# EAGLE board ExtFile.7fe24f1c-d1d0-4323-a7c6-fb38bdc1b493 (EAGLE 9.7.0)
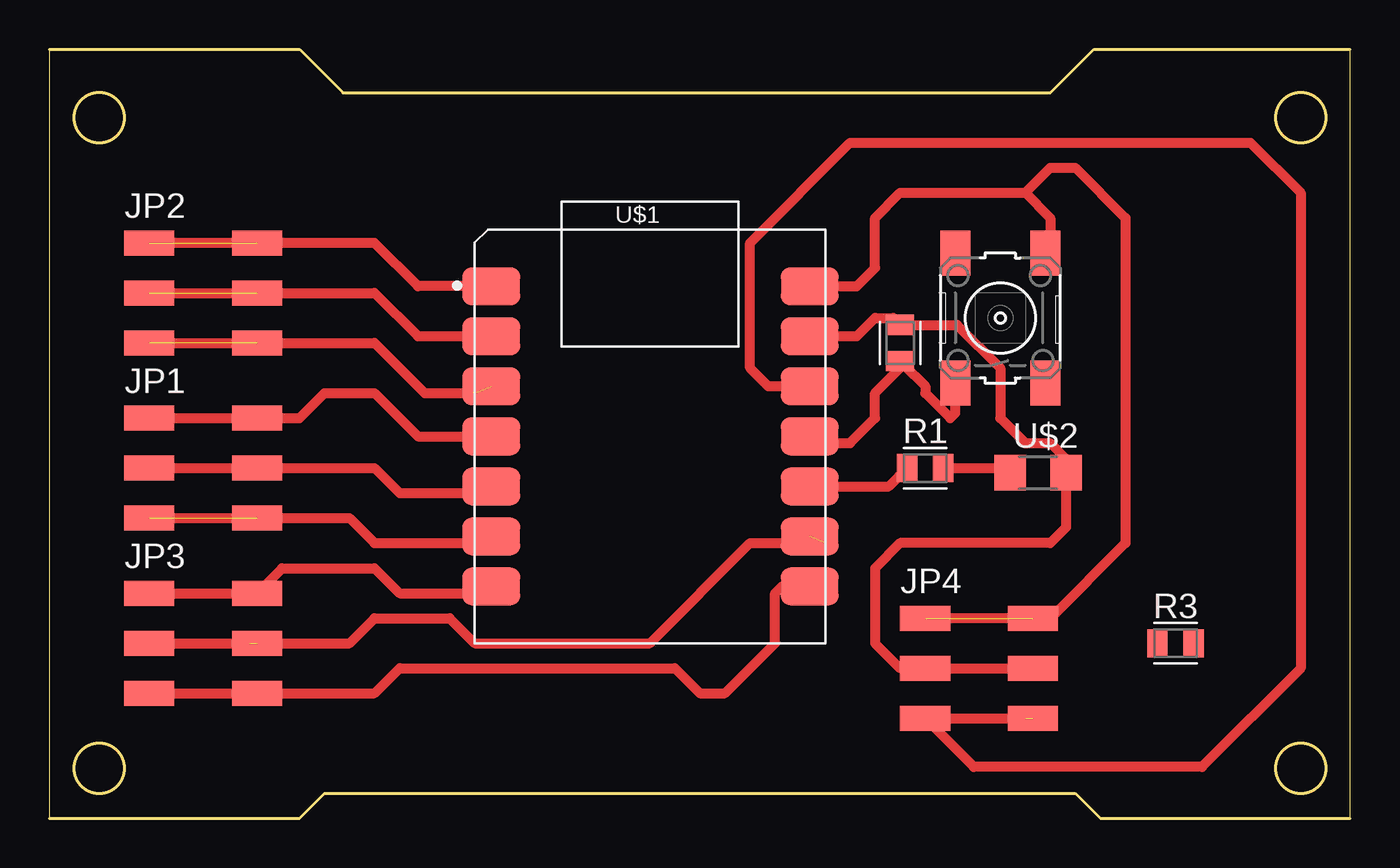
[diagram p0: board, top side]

Size 66.02 x 39.04 mm. Coordinates in mm from the lower left corner, seen from the top.
Outline: 66.02,0 66.02,39.04 53.01,39.04 50.8,36.83 14.91,36.83 12.7,39.04 0,39.04 0,0 12.7,0 13.97,1.27 52.07,1.27 53.34,0 66.02,0
Outline: circle at 2.54,35.56 radius 1.27
Outline: circle at 2.54,2.54 radius 1.27
Outline: circle at 63.5,35.56 radius 1.27
Outline: circle at 63.5,2.54 radius 1.27
Outline: circle at 63.5,35.56 radius 1.27
Outline: circle at 2.54,2.54 radius 1.27
Outline: circle at 63.5,2.54 radius 1.27
Copper layers (1*16): Top / Bottom
Stack-up Default Layer Stack: Top SilkScreen Epoxy Ink / Top SolderMask SR:Green 0.0254mm Dk 4.3 / Top Surface Finish Lead-Free 0.02mm / Top CuFoil:007 0.035mm / Dielectric-1 User Defined 1.5mm / Bottom CuFoil:007 0.035mm / Bottom Surface Finish Lead-Free 0.02mm / Bottom SolderMask SR:Green 0.0254mm Dk 4.3 / Bottom SilkScreen Epoxy Ink
Design rules: minimum drill size 0.35mm, minimum copper width 6mil, keepout clearance 0mil, drill distance 6mil, via restrict clearance 0mil, solder-mask clearance 0mil, dimension clearance 40mil, restrict clearance 0mil, copper clearance wire_polygon to wire_polygon 6mil, copper clearance wire_polygon to pad_smd 6mil, copper clearance wire_polygon to via 6mil, copper clearance pad_smd to pad_smd 6mil, copper clearance pad_smd to via 6mil, copper clearance via to via 6mil, copper clearance smd to pad (same net) 6mil, copper clearance smd to via (same net) 6mil, copper clearance smd to smd (same net) 6mil

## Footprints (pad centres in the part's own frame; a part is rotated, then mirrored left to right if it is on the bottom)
2X03SMD = smd 2.54 x 1.27: 1 -2.54,2.54; 2 2.92,2.54; 3 -2.54,0; 4 2.92,0; 5 -2.54,-2.54; 6 2.92,-2.54
RESC2012X65 = smd 1.031 x 1.42: 1 -0.919,0; 2 0.919,0
6MM_SWITCH = smd 2.286 x 1.524: 1 -3.302,2.286; 2 3.302,2.286; 3 -3.302,-2.286; 4 3.302,-2.286
XIAO_SAMD21_TAPED = smd 2.921 x 1.905: 1 0.835,18.12; 2 0.835,15.58; 3 0.835,13.04; 4 0.835,10.5; 5 0.835,7.96; 6 0.835,5.42; 7 0.835,2.88; 8 17,2.88; 9 17,5.42; 10 17,7.96; 11 17,10.5; 12 17,13.04; 13 17,15.58; 14 17,18.12
LED1206 = smd 1.6 x 1.803: 1 -1.422,0; 2 1.422,0

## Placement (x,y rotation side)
JP1  [2X03SMD]  7.62,17.78 0 top
JP2  [2X03SMD]  7.62,26.67 0 top
JP3  [2X03SMD]  7.62,8.89 0 top
JP4  [2X03SMD]  46.99,7.62 0 top
R1  [RESC2012X65]  44.45,17.78 0 top
R2  [RESC2012X65]  43.18,24.13 90 top
R3  [RESC2012X65]  57.15,8.89 0 top
S1  [6MM_SWITCH]  48.26,25.4 90 top
U$1  XIAO_SAMD21XIAO_SAMD21_TAPED  [XIAO_SAMD21_TAPED]  21.59,8.89 0 top
U$2  LED  [LED1206]  50.18,17.54 0 top

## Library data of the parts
JP1-JP4 S1 U$1 U$2 = fab
R1-R3 = Resistor; CATEGORY: Resistors; DESCRIPTION: Chip Resistor 2.00 X 1.25 X 0.65 mm body 0805(2012-METRIC) Package; PACKAGE_SIZE: 0805; PACKAGE_TYPE: Surface Mount

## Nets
3V3: JP4.5 JP4.6 U$1.12
5V: JP4.1 JP4.2 S1.4 U$1.14
D0: JP2.1 JP2.2 U$1.1
D1: JP2.3 JP2.4 U$1.2
D2: JP2.5 JP2.6 U$1.3
D3: JP1.1 JP1.2 U$1.4
D4: JP1.3 JP1.4 U$1.5
D5: JP1.5 JP1.6 U$1.6
D6: JP3.1 JP3.2 U$1.7
D7: JP3.5 JP3.6 U$1.8
D8: JP3.3 JP3.4 U$1.9
D9: R1.1 U$1.10
D10: R2.1 S1.1 U$1.11
GND: JP4.3 JP4.4 R2.2 U$1.13 U$2.2
N$6: R1.2 U$2.1

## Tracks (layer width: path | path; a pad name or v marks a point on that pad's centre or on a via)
3V3  (1 unrouted)
  Top 0.508: 49.53,5.08 JP4.5 46.91,2.62 58.5,2.62 63.5,7.62 63.5,31.75 60.96,34.29 40.64,34.29 35.56,29.21 35.56,22.86 36.49,21.93 U$1.12
5V  (1 unrouted)
  Top 0.508: U$1.14 40.98,27.01 41.91,27.94 41.91,30.48 43.18,31.75 49.53,31.75 | 49.53,31.75 50.8,30.48 50.8,28.96 S1.4 | 49.53,31.75 50.8,33.02 52.07,33.02 54.61,30.48 54.61,13.97 50.8,10.16 JP4.1
D0  (2 unrouted)
  Top 0.508: U$1.1 18.71,27.01 16.51,29.21 6.35,29.21
D1  (1 unrouted)
  Top 0.508: JP2.3 16.51,26.67 18.71,24.47 U$1.2
D2  (2 unrouted)
  Top 0.508: JP2.5 16.51,24.13 19.05,21.59 21.59,21.59
D3
  Top 0.508: JP1.1 JP1.2 12.7,20.32 13.97,21.59 16.51,21.59 18.71,19.39 U$1.4
D4
  Top 0.508: JP1.3 JP1.4 16.51,17.78 17.78,16.51 22.08,16.51 U$1.5
D5  (1 unrouted)
  Top 0.508: JP1.5 15.24,15.24 16.51,13.97 22.08,13.97 U$1.6
D6
  Top 0.508: JP3.1 JP3.2 11.81,12.7 16.51,12.7 17.78,11.43 22.08,11.43 U$1.7
D7
  Top 0.508: JP3.5 JP3.6 16.51,6.35 17.78,7.62 31.75,7.62 33.02,6.35 34.29,6.35 36.83,8.89 36.83,11.43 37.17,11.77 U$1.8
D8  (2 unrouted)
  Top 0.508: JP3.4 15.24,8.89 16.51,10.16 20.32,10.16 21.59,8.89 30.48,8.89 35.56,13.97 39.37,13.97 | JP3.3 10.16,8.89
D9
  Top 0.508: R1.1 42.6,16.85 U$1.10
D10
  Top 0.508: R2.1 43.35,23.03 | 43.35,23.03 44.45,21.94 44.45,21.59 45.72,20.32 45.97,20.57 S1.1 | U$1.11 38.93,19.05 40.64,19.05 41.91,20.32 41.91,21.59 43.35,23.03
GND
  Top 0.508: U$1.13 40.98,24.47 41.91,25.4 42.83,25.4 R2.2 46.07,25.05 48.26,22.86 48.26,20.32 49.53,19.05 50.8,19.05 51.6,18.25 U$2.2 51.6,14.77 50.8,13.97 43.18,13.97 41.91,12.7 41.91,8.89 43.18,7.62 JP4.3 JP4.4
N$6
  Top 0.508: R1.2 48.52,17.78 U$2.1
